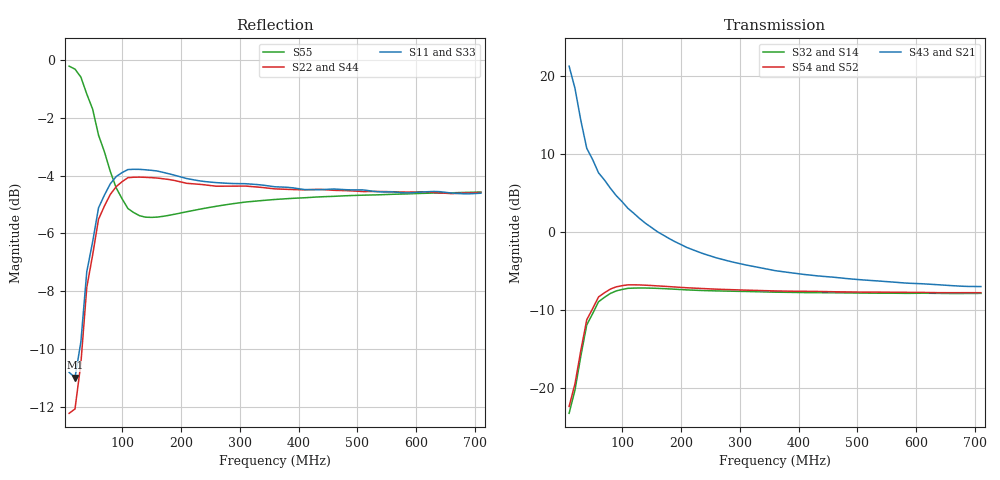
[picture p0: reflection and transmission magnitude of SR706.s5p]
!  POLYFET RF DEVICES
!  S PARAMETERS FOR
!  SR706 (EACH SIDE)
!  VDS=28, IDQ=600MA
! Date: Thu Mar 30 10:48:53 2000
!AWR Design Environment (2053) Wed Feb 04 15:53:10 2004
!freq-unit  param-type  data-format  keyword  impedance-ohms
# MHz  S  MA  R  50
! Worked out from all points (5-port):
!   71 points, 10 MHz to 710 MHz, reference 50 ohm
!   strongest paths, dB at 10 MHz, 180 MHz, 360 MHz, 540 MHz, 710 MHz:
!     S43: 21.2, -0.9, -5.0, -6.4, -7.0
!     S21: 21.2, -0.9, -5.0, -6.4, -7.0
!     S54: -22.4, -7.0, -7.6, -7.8, -7.8
!     S52: -22.4, -7.0, -7.6, -7.8, -7.8
!     S32: -23.3, -7.3, -7.8, -7.9, -7.9
!     S14: -23.3, -7.3, -7.8, -7.9, -7.9
!   lowest |S11| = -11.0 dB at 20 MHz (marker M1), VSWR 1.79, Z = 47.7 - j28.6 ohm
!   |S11| at or under -10 dB: start of sweep to 27.98 MHz
